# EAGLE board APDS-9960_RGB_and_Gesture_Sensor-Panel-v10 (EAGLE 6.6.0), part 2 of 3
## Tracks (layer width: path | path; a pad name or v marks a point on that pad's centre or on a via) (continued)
GND15  (via drill 0.38) (continued)
  other vias: 28.4,62.87 27.38,63.12 30.18,57.78 30.23,50.93 35.31,50.93 36.83,57.28 32.77,50.93 25.15,50.93 27.69,50.93 24.89,57.02 32.26,67.94 36.83,63.12 23.5,63.37
  pour Top (isolate 0.305): 22.61,68.83 37.85,68.83 37.85,48.51 22.61,48.51
  pour Bottom (isolate 0.305): 22.61,68.83 37.85,68.83 37.85,48.51 22.61,48.51
GND16  (via drill 0.38)
  Top 0.559: U17.6 44.76,63.27 44.76,63.25 44.42,62.92
  other vias: 44.15,62.87 43.13,63.12 45.92,57.78 45.97,50.93 51.05,50.93 52.58,57.28 48.51,50.93 40.89,50.93 43.43,50.93 40.64,57.02 48.01,67.94 52.58,63.12 39.24,63.37
  pour Top (isolate 0.305): 38.35,68.83 53.59,68.83 53.59,48.51 38.35,48.51
  pour Bottom (isolate 0.305): 38.35,68.83 53.59,68.83 53.59,48.51 38.35,48.51
GND17  (via drill 0.38)
  Top 0.559: U18.6 60.5,63.27 60.5,63.25 60.17,62.92
  other vias: 59.89,62.87 58.88,63.12 61.67,57.78 61.72,50.93 66.8,50.93 68.33,57.28 64.26,50.93 56.64,50.93 59.18,50.93 56.39,57.02 63.75,67.94 68.33,63.12 54.99,63.37
  pour Top (isolate 0.305): 54.1,68.83 69.34,68.83 69.34,48.51 54.1,48.51
  pour Bottom (isolate 0.305): 54.1,68.83 69.34,68.83 69.34,48.51 54.1,48.51
GND18  (via drill 0.38)
  Top 0.559: U19.6 76.25,63.27 76.25,63.25 75.92,62.92
  other vias: 75.64,62.87 74.63,63.12 77.42,57.78 77.47,50.93 82.55,50.93 84.07,57.28 80.01,50.93 72.39,50.93 74.93,50.93 72.14,57.02 79.5,67.94 84.07,63.12 70.74,63.37
  pour Top (isolate 0.305): 69.85,68.83 85.09,68.83 85.09,48.51 69.85,48.51
  pour Bottom (isolate 0.305): 69.85,68.83 85.09,68.83 85.09,48.51 69.85,48.51
GND19  (via drill 0.38)
  Top 0.559: 92.51,63.27 92,63.27 92,63.25 91.67,62.92
  other vias: 91.39,62.87 90.37,63.12 93.17,57.78 93.22,50.93 98.3,50.93 99.82,57.28 95.76,50.93 88.14,50.93 90.68,50.93 87.88,57.02 95.25,67.94 99.82,63.12 86.49,63.37
  pour Top (isolate 0.305): 85.6,68.83 100.84,68.83 100.84,48.51 85.6,48.51
  pour Bottom (isolate 0.305): 85.6,68.83 100.84,68.83 100.84,48.51 85.6,48.51
GND20  (via drill 0.38)
  Top 0.559: 108.25,63.27 107.75,63.27 107.75,63.25 107.42,62.92
  other vias: 107.14,62.87 106.12,63.12 108.92,57.78 108.97,50.93 114.05,50.93 115.57,57.28 111.51,50.93 103.89,50.93 106.43,50.93 103.63,57.02 111,67.94 115.57,63.12 102.23,63.37
  pour Top (isolate 0.305): 101.35,68.83 116.59,68.83 116.59,48.51 101.35,48.51
  pour Bottom (isolate 0.305): 101.35,68.83 116.59,68.83 116.59,48.51 101.35,48.51
GND21  (via drill 0.38)
  Top 0.559: 13.77,84.1 13.26,84.1 13.26,84.07 12.93,83.74
  other vias: 12.65,83.69 11.63,83.95 14.43,78.61 14.48,71.75 19.56,71.75 21.08,78.11 17.02,71.75 9.4,71.75 11.94,71.75 9.14,77.85 16.51,88.77 21.08,83.95 7.75,84.2
  pour Top (isolate 0.305): 6.86,89.66 22.1,89.66 22.1,69.34 6.86,69.34
  pour Bottom (isolate 0.305): 6.86,89.66 22.1,89.66 22.1,69.34 6.86,69.34
GND22  (via drill 0.38)
  Top 0.559: 29.52,84.1 29.01,84.1 29.01,84.07 28.68,83.74
  other vias: 28.4,83.69 27.38,83.95 30.18,78.61 30.23,71.75 35.31,71.75 36.83,78.11 32.77,71.75 25.15,71.75 27.69,71.75 24.89,77.85 32.26,88.77 36.83,83.95 23.5,84.2
  pour Top (isolate 0.305): 22.61,89.66 37.85,89.66 37.85,69.34 22.61,69.34
  pour Bottom (isolate 0.305): 22.61,89.66 37.85,89.66 37.85,69.34 22.61,69.34
GND23  (via drill 0.38)
  Top 0.559: U24.6 44.76,84.1 44.76,84.07 44.42,83.74
  other vias: 44.15,83.69 43.13,83.95 45.92,78.61 45.97,71.75 51.05,71.75 52.58,78.11 48.51,71.75 40.89,71.75 43.43,71.75 40.64,77.85 48.01,88.77 52.58,83.95 39.24,84.2
  pour Top (isolate 0.305): 38.35,89.66 53.59,89.66 53.59,69.34 38.35,69.34
  pour Bottom (isolate 0.305): 38.35,89.66 53.59,89.66 53.59,69.34 38.35,69.34
GND24  (via drill 0.38)
  Top 0.559: U25.6 60.5,84.1 60.5,84.07 60.17,83.74
  other vias: 59.89,83.69 58.88,83.95 61.67,78.61 61.72,71.75 66.8,71.75 68.33,78.11 64.26,71.75 56.64,71.75 59.18,71.75 56.39,77.85 63.75,88.77 68.33,83.95 54.99,84.2
  pour Top (isolate 0.305): 54.1,89.66 69.34,89.66 69.34,69.34 54.1,69.34
  pour Bottom (isolate 0.305): 54.1,89.66 69.34,89.66 69.34,69.34 54.1,69.34
GND25  (via drill 0.38)
  Top 0.559: U26.6 76.25,84.1 76.25,84.07 75.92,83.74
  other vias: 75.64,83.69 74.63,83.95 77.42,78.61 77.47,71.75 82.55,71.75 84.07,78.11 80.01,71.75 72.39,71.75 74.93,71.75 72.14,77.85 79.5,88.77 84.07,83.95 70.74,84.2
  pour Top (isolate 0.305): 69.85,89.66 85.09,89.66 85.09,69.34 69.85,69.34
  pour Bottom (isolate 0.305): 69.85,89.66 85.09,89.66 85.09,69.34 69.85,69.34
GND26  (via drill 0.38)
  Top 0.559: 92.51,84.1 92,84.1 92,84.07 91.67,83.74
  other vias: 91.39,83.69 90.37,83.95 93.17,78.61 93.22,71.75 98.3,71.75 99.82,78.11 95.76,71.75 88.14,71.75 90.68,71.75 87.88,77.85 95.25,88.77 99.82,83.95 86.49,84.2
  pour Top (isolate 0.305): 85.6,89.66 100.84,89.66 100.84,69.34 85.6,69.34
  pour Bottom (isolate 0.305): 85.6,89.66 100.84,89.66 100.84,69.34 85.6,69.34
GND27  (via drill 0.38)
  Top 0.559: 108.25,84.1 107.75,84.1 107.75,84.07 107.42,83.74
  other vias: 107.14,83.69 106.12,83.95 108.92,78.61 108.97,71.75 114.05,71.75 115.57,78.11 111.51,71.75 103.89,71.75 106.43,71.75 103.63,77.85 111,88.77 115.57,83.95 102.23,84.2
  pour Top (isolate 0.305): 101.35,89.66 116.59,89.66 116.59,69.34 101.35,69.34
  pour Bottom (isolate 0.305): 101.35,89.66 116.59,89.66 116.59,69.34 101.35,69.34
GND28  (via drill 0.38)
  Top 0.559: 13.77,104.93 13.26,104.93 13.26,104.9 12.93,104.57
  other vias: 12.65,104.52 11.63,104.78 14.43,99.44 14.48,92.58 19.56,92.58 21.08,98.93 17.02,92.58 9.4,92.58 11.94,92.58 9.14,98.68 16.51,109.6 21.08,104.78 7.75,105.03
  pour Top (isolate 0.305): 6.86,110.49 22.1,110.49 22.1,90.17 6.86,90.17
  pour Bottom (isolate 0.305): 6.86,110.49 22.1,110.49 22.1,90.17 6.86,90.17
GND29  (via drill 0.38)
  Top 0.559: 29.52,104.93 29.01,104.93 29.01,104.9 28.68,104.57
  other vias: 28.4,104.52 27.38,104.78 30.18,99.44 30.23,92.58 35.31,92.58 36.83,98.93 32.77,92.58 25.15,92.58 27.69,92.58 24.89,98.68 32.26,109.6 36.83,104.78 23.5,105.03
  pour Top (isolate 0.305): 22.61,110.49 37.85,110.49 37.85,90.17 22.61,90.17
  pour Bottom (isolate 0.305): 22.61,110.49 37.85,110.49 37.85,90.17 22.61,90.17
GND30  (via drill 0.38)
  Top 0.559: U31.6 44.76,104.93 44.76,104.9 44.42,104.57
  other vias: 44.15,104.52 43.13,104.78 45.92,99.44 45.97,92.58 51.05,92.58 52.58,98.93 48.51,92.58 40.89,92.58 43.43,92.58 40.64,98.68 48.01,109.6 52.58,104.78 39.24,105.03
  pour Top (isolate 0.305): 38.35,110.49 53.59,110.49 53.59,90.17 38.35,90.17
  pour Bottom (isolate 0.305): 38.35,110.49 53.59,110.49 53.59,90.17 38.35,90.17
GND31  (via drill 0.38)
  Top 0.559: U32.6 60.5,104.93 60.5,104.9 60.17,104.57
  other vias: 59.89,104.52 58.88,104.78 61.67,99.44 61.72,92.58 66.8,92.58 68.33,98.93 64.26,92.58 56.64,92.58 59.18,92.58 56.39,98.68 63.75,109.6 68.33,104.78 54.99,105.03
  pour Top (isolate 0.305): 54.1,110.49 69.34,110.49 69.34,90.17 54.1,90.17
  pour Bottom (isolate 0.305): 54.1,110.49 69.34,110.49 69.34,90.17 54.1,90.17
GND32  (via drill 0.38)
  Top 0.559: U33.6 76.25,104.93 76.25,104.9 75.92,104.57
  other vias: 75.64,104.52 74.63,104.78 77.42,99.44 77.47,92.58 82.55,92.58 84.07,98.93 80.01,92.58 72.39,92.58 74.93,92.58 72.14,98.68 79.5,109.6 84.07,104.78 70.74,105.03
  pour Top (isolate 0.305): 69.85,110.49 85.09,110.49 85.09,90.17 69.85,90.17
  pour Bottom (isolate 0.305): 69.85,110.49 85.09,110.49 85.09,90.17 69.85,90.17
GND33  (via drill 0.38)
  Top 0.559: 92.51,104.93 92,104.93 92,104.9 91.67,104.57
  other vias: 91.39,104.52 90.37,104.78 93.17,99.44 93.22,92.58 98.3,92.58 99.82,98.93 95.76,92.58 88.14,92.58 90.68,92.58 87.88,98.68 95.25,109.6 99.82,104.78 86.49,105.03
  pour Top (isolate 0.305): 85.6,110.49 100.84,110.49 100.84,90.17 85.6,90.17
  pour Bottom (isolate 0.305): 85.6,110.49 100.84,110.49 100.84,90.17 85.6,90.17
GND34  (via drill 0.38)
  Top 0.559: 108.25,104.93 107.75,104.93 107.75,104.9 107.42,104.57
  other vias: 107.14,104.52 106.12,104.78 108.92,99.44 108.97,92.58 114.05,92.58 115.57,98.93 111.51,92.58 103.89,92.58 106.43,92.58 103.63,98.68 111,109.6 115.57,104.78 102.23,105.03
  pour Top (isolate 0.305): 101.35,110.49 116.59,110.49 116.59,90.17 101.35,90.17
  pour Bottom (isolate 0.305): 101.35,110.49 116.59,110.49 116.59,90.17 101.35,90.17
INT  (via drill 0.38)
  Top 0.305: U1.2 16.28,22.58 16.51,22.35 v16.51,21.59 16.51,21.12 R1.1
  Bottom 0.305: JP1.6 20.83,14.48 18.29,17.02 18.29,19.81 v16.51,21.59
INT1  (via drill 0.38)
  Top 0.305: U2.2 32.03,22.58 32.26,22.35 v32.26,21.59 32.26,21.12 R5.1
  Bottom 0.305: JP2.6 36.58,14.48 34.04,17.02 34.04,19.81 v32.26,21.59
INT2  (via drill 0.38)
  Top 0.305: U3.2 47.77,22.58 48.01,22.35 v48.01,21.59 48.01,21.12 R9.1
  Bottom 0.305: JP3.6 52.32,14.48 49.78,17.02 49.78,19.81 v48.01,21.59
INT3  (via drill 0.38)
  Top 0.305: U4.2 63.52,22.58 63.75,22.35 v63.75,21.59 63.75,21.12 R13.1
  Bottom 0.305: JP4.6 68.07,14.48 65.53,17.02 65.53,19.81 v63.75,21.59
INT4  (via drill 0.38)
  Top 0.305: U5.2 79.27,22.58 79.5,22.35 v79.5,21.59 79.5,21.12 R17.1
  Bottom 0.305: JP5.6 83.82,14.48 81.28,17.02 81.28,19.81 v79.5,21.59
INT5  (via drill 0.38)
  Top 0.305: U6.2 95.02,22.58 95.25,22.35 v95.25,21.59 95.25,21.12 R21.1
  Bottom 0.305: JP6.6 99.57,14.48 97.03,17.02 97.03,19.81 v95.25,21.59
INT6  (via drill 0.38)
  Top 0.305: U7.2 110.77,22.58 111,22.35 v111,21.59 111,21.12 R25.1
  Bottom 0.305: JP7.6 115.32,14.48 112.78,17.02 112.78,19.81 v111,21.59
INT7  (via drill 0.38)
  Top 0.305: U8.2 16.28,43.41 16.51,43.18 v16.51,42.42 16.51,41.95 R29.1
  Bottom 0.305: JP8.6 20.83,35.31 18.29,37.85 18.29,40.64 v16.51,42.42
INT8  (via drill 0.38)
  Top 0.305: U9.2 32.03,43.41 32.26,43.18 v32.26,42.42 32.26,41.95 R33.1
  Bottom 0.305: JP9.6 36.58,35.31 34.04,37.85 34.04,40.64 v32.26,42.42
INT9  (via drill 0.38)
  Top 0.305: U10.2 47.77,43.41 48.01,43.18 v48.01,42.42 48.01,41.95 R37.1
  Bottom 0.305: JP10.6 52.32,35.31 49.78,37.85 49.78,40.64 v48.01,42.42
INT10  (via drill 0.38)
  Top 0.305: U11.2 63.52,43.41 63.75,43.18 v63.75,42.42 63.75,41.95 R41.1
  Bottom 0.305: JP11.6 68.07,35.31 65.53,37.85 65.53,40.64 v63.75,42.42
INT11  (via drill 0.38)
  Top 0.305: U12.2 79.27,43.41 79.5,43.18 v79.5,42.42 79.5,41.95 R45.1
  Bottom 0.305: JP12.6 83.82,35.31 81.28,37.85 81.28,40.64 v79.5,42.42
INT12  (via drill 0.38)
  Top 0.305: U13.2 95.02,43.41 95.25,43.18 v95.25,42.42 95.25,41.95 R49.1
  Bottom 0.305: JP13.6 99.57,35.31 97.03,37.85 97.03,40.64 v95.25,42.42
INT13  (via drill 0.38)
  Top 0.305: U14.2 110.77,43.41 111,43.18 v111,42.42 111,41.95 R53.1
  Bottom 0.305: JP14.6 115.32,35.31 112.78,37.85 112.78,40.64 v111,42.42
INT14  (via drill 0.38)
  Top 0.305: U15.2 16.28,64.24 16.51,64.01 v16.51,63.25 16.51,62.78 R57.1
  Bottom 0.305: JP15.6 20.83,56.13 18.29,58.67 18.29,61.47 v16.51,63.25
INT15  (via drill 0.38)
  Top 0.305: U16.2 32.03,64.24 32.26,64.01 v32.26,63.25 32.26,62.78 R61.1
  Bottom 0.305: JP16.6 36.58,56.13 34.04,58.67 34.04,61.47 v32.26,63.25
INT16  (via drill 0.38)
  Top 0.305: U17.2 47.77,64.24 48.01,64.01 v48.01,63.25 48.01,62.78 R65.1
  Bottom 0.305: JP17.6 52.32,56.13 49.78,58.67 49.78,61.47 v48.01,63.25
INT17  (via drill 0.38)
  Top 0.305: U18.2 63.52,64.24 63.75,64.01 v63.75,63.25 63.75,62.78 R69.1
  Bottom 0.305: JP18.6 68.07,56.13 65.53,58.67 65.53,61.47 v63.75,63.25
INT18  (via drill 0.38)
  Top 0.305: U19.2 79.27,64.24 79.5,64.01 v79.5,63.25 79.5,62.78 R73.1
  Bottom 0.305: JP19.6 83.82,56.13 81.28,58.67 81.28,61.47 v79.5,63.25
INT19  (via drill 0.38)
  Top 0.305: U20.2 95.02,64.24 95.25,64.01 v95.25,63.25 95.25,62.78 R77.1
  Bottom 0.305: JP20.6 99.57,56.13 97.03,58.67 97.03,61.47 v95.25,63.25
INT20  (via drill 0.38)
  Top 0.305: U21.2 110.77,64.24 111,64.01 v111,63.25 111,62.78 R81.1
  Bottom 0.305: JP21.6 115.32,56.13 112.78,58.67 112.78,61.47 v111,63.25
INT21  (via drill 0.38)
  Top 0.305: U22.2 16.28,85.07 16.51,84.84 v16.51,84.07 16.51,83.61 R85.1
  Bottom 0.305: JP22.6 20.83,76.96 18.29,79.5 18.29,82.3 v16.51,84.07
INT22  (via drill 0.38)
  Top 0.305: U23.2 32.03,85.07 32.26,84.84 v32.26,84.07 32.26,83.61 R89.1
  Bottom 0.305: JP23.6 36.58,76.96 34.04,79.5 34.04,82.3 v32.26,84.07
INT23  (via drill 0.38)
  Top 0.305: U24.2 47.77,85.07 48.01,84.84 v48.01,84.07 48.01,83.61 R93.1
  Bottom 0.305: JP24.6 52.32,76.96 49.78,79.5 49.78,82.3 v48.01,84.07
INT24  (via drill 0.38)
  Top 0.305: U25.2 63.52,85.07 63.75,84.84 v63.75,84.07 63.75,83.61 R97.1
  Bottom 0.305: JP25.6 68.07,76.96 65.53,79.5 65.53,82.3 v63.75,84.07
INT25  (via drill 0.38)
  Top 0.305: U26.2 79.27,85.07 79.5,84.84 v79.5,84.07 79.5,83.61 R101.1
  Bottom 0.305: JP26.6 83.82,76.96 81.28,79.5 81.28,82.3 v79.5,84.07
INT26  (via drill 0.38)
  Top 0.305: U27.2 95.02,85.07 95.25,84.84 v95.25,84.07 95.25,83.61 R105.1
  Bottom 0.305: JP27.6 99.57,76.96 97.03,79.5 97.03,82.3 v95.25,84.07
INT27  (via drill 0.38)
  Top 0.305: U28.2 110.77,85.07 111,84.84 v111,84.07 111,83.61 R109.1
  Bottom 0.305: JP28.6 115.32,76.96 112.78,79.5 112.78,82.3 v111,84.07
INT28  (via drill 0.38)
  Top 0.305: U29.2 16.28,105.89 16.51,105.66 v16.51,104.9 16.51,104.43 R113.1
  Bottom 0.305: JP29.6 20.83,97.79 18.29,100.33 18.29,103.12 v16.51,104.9
INT29  (via drill 0.38)
  Top 0.305: U30.2 32.03,105.89 32.26,105.66 v32.26,104.9 32.26,104.43 R117.1
  Bottom 0.305: JP30.6 36.58,97.79 34.04,100.33 34.04,103.12 v32.26,104.9
INT30  (via drill 0.38)
  Top 0.305: U31.2 47.77,105.89 48.01,105.66 v48.01,104.9 48.01,104.43 R121.1
  Bottom 0.305: JP31.6 52.32,97.79 49.78,100.33 49.78,103.12 v48.01,104.9
INT31  (via drill 0.38)
  Top 0.305: U32.2 63.52,105.89 63.75,105.66 v63.75,104.9 63.75,104.43 R125.1
  Bottom 0.305: JP32.6 68.07,97.79 65.53,100.33 65.53,103.12 v63.75,104.9
INT32  (via drill 0.38)
  Top 0.305: U33.2 79.27,105.89 79.5,105.66 v79.5,104.9 79.5,104.43 R129.1
  Bottom 0.305: JP33.6 83.82,97.79 81.28,100.33 81.28,103.12 v79.5,104.9
INT33  (via drill 0.38)
  Top 0.305: U34.2 95.02,105.89 95.25,105.66 v95.25,104.9 95.25,104.43 R133.1
  Bottom 0.305: JP34.6 99.57,97.79 97.03,100.33 97.03,103.12 v95.25,104.9
INT34  (via drill 0.38)
  Top 0.305: U35.2 110.77,105.89 111,105.66 v111,104.9 111,104.43 R137.1
  Bottom 0.305: JP35.6 115.32,97.79 112.78,100.33 112.78,103.12 v111,104.9
N$1
  Top 0.305: R2.2 15.75,16 16,15.75 19.3,15.75 19.56,16 19.56,16.51 19.89,16.84 SJ1.3
N$2
  Top 0.305: SJ1.1 18.32,18.47 R3.2
N$4
  Top 0.559: U1.4 U1.3
N$5
  Top 0.305: R6.2 31.5,16 31.75,15.75 35.05,15.75 35.31,16 35.31,16.51 35.64,16.84 SJ3.3
N$6
  Top 0.305: SJ3.1 34.07,18.47 R8.2
N$7
  Top 0.559: U2.4 U2.3
N$8
  Top 0.305: R10.2 47.24,16 47.5,15.75 50.8,15.75 51.05,16 51.05,16.51 51.38,16.84 SJ5.3
N$9
  Top 0.305: SJ5.1 49.82,18.47 R12.2
N$10
  Top 0.559: U3.4 U3.3
N$11
  Top 0.305: R14.2 62.99,16 63.25,15.75 66.55,15.75 66.8,16 66.8,16.51 67.13,16.84 SJ7.3
N$12
  Top 0.305: SJ7.1 65.57,18.47 R16.2
N$13
  Top 0.559: U4.4 U4.3
N$14
  Top 0.305: R18.2 78.74,16 78.99,15.75 82.3,15.75 82.55,16 82.55,16.51 82.88,16.84 SJ9.3
N$15
  Top 0.305: SJ9.1 81.32,18.47 R20.2
N$16
  Top 0.559: U5.4 U5.3
N$17
  Top 0.305: R22.2 94.49,16 94.74,15.75 98.04,15.75 98.3,16 98.3,16.51 98.63,16.84 SJ11.3
N$18
  Top 0.305: SJ11.1 97.06,18.47 R24.2
N$19
  Top 0.559: U6.4 U6.3
N$20
  Top 0.305: R26.2 110.24,16 110.49,15.75 113.79,15.75 114.05,16 114.05,16.51 114.38,16.84 SJ13.3
N$21
  Top 0.305: SJ13.1 112.81,18.47 R28.2
N$22
  Top 0.559: U7.4 U7.3
N$23
  Top 0.305: R30.2 15.75,36.83 16,36.58 19.3,36.58 19.56,36.83 19.56,37.34 19.89,37.67 SJ15.3
N$24
  Top 0.305: SJ15.1 18.32,39.29 R32.2
N$25
  Top 0.559: U8.4 U8.3
N$26
  Top 0.305: R34.2 31.5,36.83 31.75,36.58 35.05,36.58 35.31,36.83 35.31,37.34 35.64,37.67 SJ17.3
N$27
  Top 0.305: SJ17.1 34.07,39.29 R36.2
N$28
  Top 0.559: U9.4 U9.3
N$29
  Top 0.305: R38.2 47.24,36.83 47.5,36.58 50.8,36.58 51.05,36.83 51.05,37.34 51.38,37.67 SJ19.3
N$30
  Top 0.305: SJ19.1 49.82,39.29 R40.2
N$31
  Top 0.559: U10.4 U10.3
N$32
  Top 0.305: R42.2 62.99,36.83 63.25,36.58 66.55,36.58 66.8,36.83 66.8,37.34 67.13,37.67 SJ21.3
N$33
  Top 0.305: SJ21.1 65.57,39.29 R44.2
N$34
  Top 0.559: U11.4 U11.3
N$35
  Top 0.305: R46.2 78.74,36.83 78.99,36.58 82.3,36.58 82.55,36.83 82.55,37.34 82.88,37.67 SJ23.3
N$36
  Top 0.305: SJ23.1 81.32,39.29 R48.2
N$37
  Top 0.559: U12.4 U12.3
N$38
  Top 0.305: R50.2 94.49,36.83 94.74,36.58 98.04,36.58 98.3,36.83 98.3,37.34 98.63,37.67 SJ25.3
N$39
  Top 0.305: SJ25.1 97.06,39.29 R52.2
N$40
  Top 0.559: U13.4 U13.3
N$41
  Top 0.305: R54.2 110.24,36.83 110.49,36.58 113.79,36.58 114.05,36.83 114.05,37.34 114.38,37.67 SJ27.3
N$42
  Top 0.305: SJ27.1 112.81,39.29 R56.2
N$43
  Top 0.559: U14.4 U14.3
N$44
  Top 0.305: R58.2 15.75,57.66 16,57.4 19.3,57.4 19.56,57.66 19.56,58.17 19.89,58.5 SJ29.3
N$45
  Top 0.305: SJ29.1 18.32,60.12 R60.2
N$46
  Top 0.559: U15.4 U15.3
N$47
  Top 0.305: R62.2 31.5,57.66 31.75,57.4 35.05,57.4 35.31,57.66 35.31,58.17 35.64,58.5 SJ31.3
N$48
  Top 0.305: SJ31.1 34.07,60.12 R64.2
N$49
  Top 0.559: U16.4 U16.3
N$50
  Top 0.305: R66.2 47.24,57.66 47.5,57.4 50.8,57.4 51.05,57.66 51.05,58.17 51.38,58.5 SJ33.3
N$51
  Top 0.305: SJ33.1 49.82,60.12 R68.2
N$52
  Top 0.559: U17.4 U17.3
N$53
  Top 0.305: R70.2 62.99,57.66 63.25,57.4 66.55,57.4 66.8,57.66 66.8,58.17 67.13,58.5 SJ35.3
N$54
  Top 0.305: SJ35.1 65.57,60.12 R72.2
N$55
  Top 0.559: U18.4 U18.3
N$56
  Top 0.305: R74.2 78.74,57.66 78.99,57.4 82.3,57.4 82.55,57.66 82.55,58.17 82.88,58.5 SJ37.3
N$57
  Top 0.305: SJ37.1 81.32,60.12 R76.2
N$58
  Top 0.559: U19.4 U19.3
N$59
  Top 0.305: R78.2 94.49,57.66 94.74,57.4 98.04,57.4 98.3,57.66 98.3,58.17 98.63,58.5 SJ39.3
N$60
  Top 0.305: SJ39.1 97.06,60.12 R80.2
N$61
  Top 0.559: U20.4 U20.3
N$62
  Top 0.305: R82.2 110.24,57.66 110.49,57.4 113.79,57.4 114.05,57.66 114.05,58.17 114.38,58.5 SJ41.3
N$63
  Top 0.305: SJ41.1 112.81,60.12 R84.2
N$64
  Top 0.559: U21.4 U21.3
N$65
  Top 0.305: R86.2 15.75,78.49 16,78.23 19.3,78.23 19.56,78.49 19.56,78.99 19.89,79.32 SJ43.3
N$66
  Top 0.305: SJ43.1 18.32,80.95 R88.2
N$67
  Top 0.559: U22.4 U22.3
N$68
  Top 0.305: R90.2 31.5,78.49 31.75,78.23 35.05,78.23 35.31,78.49 35.31,78.99 35.64,79.32 SJ45.3
N$69
  Top 0.305: SJ45.1 34.07,80.95 R92.2
N$70
  Top 0.559: U23.4 U23.3
N$71
  Top 0.305: R94.2 47.24,78.49 47.5,78.23 50.8,78.23 51.05,78.49 51.05,78.99 51.38,79.32 SJ47.3
N$72
  Top 0.305: SJ47.1 49.82,80.95 R96.2
N$73
  Top 0.559: U24.4 U24.3
N$74
  Top 0.305: R98.2 62.99,78.49 63.25,78.23 66.55,78.23 66.8,78.49 66.8,78.99 67.13,79.32 SJ49.3
N$75
  Top 0.305: SJ49.1 65.57,80.95 R100.2
N$76
  Top 0.559: U25.4 U25.3
N$77
  Top 0.305: R102.2 78.74,78.49 78.99,78.23 82.3,78.23 82.55,78.49 82.55,78.99 82.88,79.32 SJ51.3
N$78
  Top 0.305: SJ51.1 81.32,80.95 R104.2
N$79
  Top 0.559: U26.4 U26.3
N$80
  Top 0.305: R106.2 94.49,78.49 94.74,78.23 98.04,78.23 98.3,78.49 98.3,78.99 98.63,79.32 SJ53.3
N$81
  Top 0.305: SJ53.1 97.06,80.95 R108.2
N$82
  Top 0.559: U27.4 U27.3
N$83
  Top 0.305: R110.2 110.24,78.49 110.49,78.23 113.79,78.23 114.05,78.49 114.05,78.99 114.38,79.32 SJ55.3
N$84
  Top 0.305: SJ55.1 112.81,80.95 R112.2
N$85
  Top 0.559: U28.4 U28.3
N$86
  Top 0.305: R114.2 15.75,99.31 16,99.06 19.3,99.06 19.56,99.31 19.56,99.82 19.89,100.15 SJ57.3
N$87
  Top 0.305: SJ57.1 18.32,101.78 R116.2
N$88
  Top 0.559: U29.4 U29.3
N$89
  Top 0.305: R118.2 31.5,99.31 31.75,99.06 35.05,99.06 35.31,99.31 35.31,99.82 35.64,100.15 SJ59.3
N$90
  Top 0.305: SJ59.1 34.07,101.78 R120.2
N$91
  Top 0.559: U30.4 U30.3
N$92
  Top 0.305: R122.2 47.24,99.31 47.5,99.06 50.8,99.06 51.05,99.31 51.05,99.82 51.38,100.15 SJ61.3
N$93
  Top 0.305: SJ61.1 49.82,101.78 R124.2
N$94
  Top 0.559: U31.4 U31.3
N$95
  Top 0.305: R126.2 62.99,99.31 63.25,99.06 66.55,99.06 66.8,99.31 66.8,99.82 67.13,100.15 SJ63.3
N$96
  Top 0.305: SJ63.1 65.57,101.78 R128.2
N$97
  Top 0.559: U32.4 U32.3
N$98
  Top 0.305: R130.2 78.74,99.31 78.99,99.06 82.3,99.06 82.55,99.31 82.55,99.82 82.88,100.15 SJ65.3
N$99
  Top 0.305: SJ65.1 81.32,101.78 R132.2
N$100
  Top 0.559: U33.4 U33.3
N$101
  Top 0.305: R134.2 94.49,99.31 94.74,99.06 98.04,99.06 98.3,99.31 98.3,99.82 98.63,100.15 SJ67.3
N$102
  Top 0.305: SJ67.1 97.06,101.78 R136.2
N$103
  Top 0.559: U34.4 U34.3
N$104
  Top 0.305: R138.2 110.24,99.31 110.49,99.06 113.79,99.06 114.05,99.31 114.05,99.82 114.38,100.15 SJ69.3
N$105
  Top 0.305: SJ69.1 112.81,101.78 R140.2
N$106
  Top 0.559: U35.4 U35.3
SCL  (via drill 0.38)
  Top 0.305: U1.7 12.78,22.58 v12.7,22.5 | R3.1 17.06,16.8 v17.02,16.76
  Bottom 0.305: JP1.5 18.29,15.49 v17.02,16.76 15.24,18.54 15.24,24.13 15.39,24.28 15.39,25.15 14.86,25.68 13.23,25.68 12.7,25.15 v12.7,22.5
SCL1  (via drill 0.38)
  Top 0.305: U2.7 28.53,22.58 v28.45,22.5 | R8.1 32.8,16.8 v32.77,16.76
  Bottom 0.305: JP2.5 34.04,15.49 v32.77,16.76 30.99,18.54 30.99,24.13 31.14,24.28 31.14,25.15 30.61,25.68 28.98,25.68 28.45,25.15 v28.45,22.5
SCL2  (via drill 0.38)
  Top 0.305: U3.7 44.27,22.58 v44.2,22.5 | R12.1 48.55,16.8 v48.51,16.76
  Bottom 0.305: JP3.5 49.78,15.49 v48.51,16.76 46.74,18.54 46.74,24.13 46.89,24.28 46.89,25.15 46.35,25.68 44.73,25.68 44.2,25.15 v44.2,22.5
SCL3  (via drill 0.38)
  Top 0.305: U4.7 60.02,22.58 v59.94,22.5 | R16.1 64.3,16.8 v64.26,16.76
  Bottom 0.305: JP4.5 65.53,15.49 v64.26,16.76 62.48,18.54 62.48,24.13 62.64,24.28 62.64,25.15 62.1,25.68 60.48,25.68 59.94,25.15 v59.94,22.5
SCL4  (via drill 0.38)
  Top 0.305: U5.7 75.77,22.58 v75.69,22.5 | R20.1 80.05,16.8 v80.01,16.76
  Bottom 0.305: JP5.5 81.28,15.49 v80.01,16.76 78.23,18.54 78.23,24.13 78.38,24.28 78.38,25.15 77.85,25.68 76.22,25.68 75.69,25.15 v75.69,22.5
SCL5  (via drill 0.38)
  Top 0.305: U6.7 91.52,22.58 v91.44,22.5 | R24.1 95.8,16.8 v95.76,16.76
  Bottom 0.305: JP6.5 97.03,15.49 v95.76,16.76 93.98,18.54 93.98,24.13 94.13,24.28 94.13,25.15 93.6,25.68 91.97,25.68 91.44,25.15 v91.44,22.5
SCL6  (via drill 0.38)
  Top 0.305: U7.7 107.27,22.58 v107.19,22.5 | R28.1 111.55,16.8 v111.51,16.76
  Bottom 0.305: JP7.5 112.78,15.49 v111.51,16.76 109.73,18.54 109.73,24.13 109.88,24.28 109.88,25.15 109.35,25.68 107.72,25.68 107.19,25.15 v107.19,22.5
SCL7  (via drill 0.38)
  Top 0.305: U8.7 12.78,43.41 v12.7,43.33 | R32.1 17.06,37.63 v17.02,37.59
  Bottom 0.305: JP8.5 18.29,36.32 v17.02,37.59 15.24,39.37 15.24,44.96 15.39,45.11 15.39,45.97 14.86,46.51 13.23,46.51 12.7,45.97 v12.7,43.33
SCL8  (via drill 0.38)
  Top 0.305: U9.7 28.53,43.41 v28.45,43.33 | R36.1 32.8,37.63 v32.77,37.59
  Bottom 0.305: JP9.5 34.04,36.32 v32.77,37.59 30.99,39.37 30.99,44.96 31.14,45.11 31.14,45.97 30.61,46.51 28.98,46.51 28.45,45.97 v28.45,43.33
SCL9  (via drill 0.38)
  Top 0.305: U10.7 44.27,43.41 v44.2,43.33 | R40.1 48.55,37.63 v48.51,37.59
  Bottom 0.305: JP10.5 49.78,36.32 v48.51,37.59 46.74,39.37 46.74,44.96 46.89,45.11 46.89,45.97 46.35,46.51 44.73,46.51 44.2,45.97 v44.2,43.33
SCL10  (via drill 0.38)
  Top 0.305: U11.7 60.02,43.41 v59.94,43.33 | R44.1 64.3,37.63 v64.26,37.59
  Bottom 0.305: JP11.5 65.53,36.32 v64.26,37.59 62.48,39.37 62.48,44.96 62.64,45.11 62.64,45.97 62.1,46.51 60.48,46.51 59.94,45.97 v59.94,43.33
SCL11  (via drill 0.38)
  Top 0.305: U12.7 75.77,43.41 v75.69,43.33 | R48.1 80.05,37.63 v80.01,37.59
  Bottom 0.305: JP12.5 81.28,36.32 v80.01,37.59 78.23,39.37 78.23,44.96 78.38,45.11 78.38,45.97 77.85,46.51 76.22,46.51 75.69,45.97 v75.69,43.33
SCL12  (via drill 0.38)
  Top 0.305: U13.7 91.52,43.41 v91.44,43.33 | R52.1 95.8,37.63 v95.76,37.59
  Bottom 0.305: JP13.5 97.03,36.32 v95.76,37.59 93.98,39.37 93.98,44.96 94.13,45.11 94.13,45.97 93.6,46.51 91.97,46.51 91.44,45.97 v91.44,43.33
SCL13  (via drill 0.38)
  Top 0.305: U14.7 107.27,43.41 v107.19,43.33 | R56.1 111.55,37.63 v111.51,37.59
  Bottom 0.305: JP14.5 112.78,36.32 v111.51,37.59 109.73,39.37 109.73,44.96 109.88,45.11 109.88,45.97 109.35,46.51 107.72,46.51 107.19,45.97 v107.19,43.33
SCL14  (via drill 0.38)
  Top 0.305: U15.7 12.78,64.24 v12.7,64.16 | R60.1 17.06,58.46 v17.02,58.42
  Bottom 0.305: JP15.5 18.29,57.15 v17.02,58.42 15.24,60.2 15.24,65.79 15.39,65.94 15.39,66.8 14.86,67.33 13.23,67.33 12.7,66.8 v12.7,64.16
SCL15  (via drill 0.38)
  Top 0.305: U16.7 28.53,64.24 v28.45,64.16 | R64.1 32.8,58.46 v32.77,58.42
  Bottom 0.305: JP16.5 34.04,57.15 v32.77,58.42 30.99,60.2 30.99,65.79 31.14,65.94 31.14,66.8 30.61,67.33 28.98,67.33 28.45,66.8 v28.45,64.16
SCL16  (via drill 0.38)
  Top 0.305: U17.7 44.27,64.24 v44.2,64.16 | R68.1 48.55,58.46 v48.51,58.42
  Bottom 0.305: JP17.5 49.78,57.15 v48.51,58.42 46.74,60.2 46.74,65.79 46.89,65.94 46.89,66.8 46.35,67.33 44.73,67.33 44.2,66.8 v44.2,64.16
SCL17  (via drill 0.38)
  Top 0.305: U18.7 60.02,64.24 v59.94,64.16 | R72.1 64.3,58.46 v64.26,58.42
  Bottom 0.305: JP18.5 65.53,57.15 v64.26,58.42 62.48,60.2 62.48,65.79 62.64,65.94 62.64,66.8 62.1,67.33 60.48,67.33 59.94,66.8 v59.94,64.16
SCL18  (via drill 0.38)
  Top 0.305: U19.7 75.77,64.24 v75.69,64.16 | R76.1 80.05,58.46 v80.01,58.42
  Bottom 0.305: JP19.5 81.28,57.15 v80.01,58.42 78.23,60.2 78.23,65.79 78.38,65.94 78.38,66.8 77.85,67.33 76.22,67.33 75.69,66.8 v75.69,64.16
SCL19  (via drill 0.38)
  Top 0.305: U20.7 91.52,64.24 v91.44,64.16 | R80.1 95.8,58.46 v95.76,58.42
  Bottom 0.305: JP20.5 97.03,57.15 v95.76,58.42 93.98,60.2 93.98,65.79 94.13,65.94 94.13,66.8 93.6,67.33 91.97,67.33 91.44,66.8 v91.44,64.16
SCL20  (via drill 0.38)
  Top 0.305: U21.7 107.27,64.24 v107.19,64.16 | R84.1 111.55,58.46 v111.51,58.42
  Bottom 0.305: JP21.5 112.78,57.15 v111.51,58.42 109.73,60.2 109.73,65.79 109.88,65.94 109.88,66.8 109.35,67.33 107.72,67.33 107.19,66.8 v107.19,64.16
SCL21  (via drill 0.38)
  Top 0.305: U22.7 12.78,85.07 v12.7,84.99 | R88.1 17.06,79.29 v17.02,79.25
  Bottom 0.305: JP22.5 18.29,77.98 v17.02,79.25 15.24,81.03 15.24,86.61 15.39,86.77 15.39,87.63 14.86,88.16 13.23,88.16 12.7,87.63 v12.7,84.99
SCL22  (via drill 0.38)
  Top 0.305: U23.7 28.53,85.07 v28.45,84.99 | R92.1 32.8,79.29 v32.77,79.25
  Bottom 0.305: JP23.5 34.04,77.98 v32.77,79.25 30.99,81.03 30.99,86.61 31.14,86.77 31.14,87.63 30.61,88.16 28.98,88.16 28.45,87.63 v28.45,84.99
SCL23  (via drill 0.38)
  Top 0.305: U24.7 44.27,85.07 v44.2,84.99 | R96.1 48.55,79.29 v48.51,79.25
  Bottom 0.305: JP24.5 49.78,77.98 v48.51,79.25 46.74,81.03 46.74,86.61 46.89,86.77 46.89,87.63 46.35,88.16 44.73,88.16 44.2,87.63 v44.2,84.99
SCL24  (via drill 0.38)
  Top 0.305: U25.7 60.02,85.07 v59.94,84.99 | R100.1 64.3,79.29 v64.26,79.25
  Bottom 0.305: JP25.5 65.53,77.98 v64.26,79.25 62.48,81.03 62.48,86.61 62.64,86.77 62.64,87.63 62.1,88.16 60.48,88.16 59.94,87.63 v59.94,84.99
SCL25  (via drill 0.38)
  Top 0.305: U26.7 75.77,85.07 v75.69,84.99 | R104.1 80.05,79.29 v80.01,79.25
  Bottom 0.305: JP26.5 81.28,77.98 v80.01,79.25 78.23,81.03 78.23,86.61 78.38,86.77 78.38,87.63 77.85,88.16 76.22,88.16 75.69,87.63 v75.69,84.99
SCL26  (via drill 0.38)
  Top 0.305: U27.7 91.52,85.07 v91.44,84.99 | R108.1 95.8,79.29 v95.76,79.25
  Bottom 0.305: JP27.5 97.03,77.98 v95.76,79.25 93.98,81.03 93.98,86.61 94.13,86.77 94.13,87.63 93.6,88.16 91.97,88.16 91.44,87.63 v91.44,84.99
SCL27  (via drill 0.38)
  Top 0.305: U28.7 107.27,85.07 v107.19,84.99 | R112.1 111.55,79.29 v111.51,79.25
  Bottom 0.305: JP28.5 112.78,77.98 v111.51,79.25 109.73,81.03 109.73,86.61 109.88,86.77 109.88,87.63 109.35,88.16 107.72,88.16 107.19,87.63 v107.19,84.99
SCL28  (via drill 0.38)
  Top 0.305: U29.7 12.78,105.89 v12.7,105.82 | R116.1 17.06,100.11 v17.02,100.08
  Bottom 0.305: JP29.5 18.29,98.81 v17.02,100.08 15.24,101.85 15.24,107.44 15.39,107.59 15.39,108.46 14.86,108.99 13.23,108.99 12.7,108.46 v12.7,105.82
SCL29  (via drill 0.38)
  Top 0.305: U30.7 28.53,105.89 v28.45,105.82 | R120.1 32.8,100.11 v32.77,100.08
  Bottom 0.305: JP30.5 34.04,98.81 v32.77,100.08 30.99,101.85 30.99,107.44 31.14,107.59 31.14,108.46 30.61,108.99 28.98,108.99 28.45,108.46 v28.45,105.82
SCL30  (via drill 0.38)
  Top 0.305: U31.7 44.27,105.89 v44.2,105.82 | R124.1 48.55,100.11 v48.51,100.08
  Bottom 0.305: JP31.5 49.78,98.81 v48.51,100.08 46.74,101.85 46.74,107.44 46.89,107.59 46.89,108.46 46.35,108.99 44.73,108.99 44.2,108.46 v44.2,105.82
SCL31  (via drill 0.38)
  Top 0.305: U32.7 60.02,105.89 v59.94,105.82 | R128.1 64.3,100.11 v64.26,100.08
  Bottom 0.305: JP32.5 65.53,98.81 v64.26,100.08 62.48,101.85 62.48,107.44 62.64,107.59 62.64,108.46 62.1,108.99 60.48,108.99 59.94,108.46 v59.94,105.82
SCL32  (via drill 0.38)
  Top 0.305: U33.7 75.77,105.89 v75.69,105.82 | R132.1 80.05,100.11 v80.01,100.08
  Bottom 0.305: JP33.5 81.28,98.81 v80.01,100.08 78.23,101.85 78.23,107.44 78.38,107.59 78.38,108.46 77.85,108.99 76.22,108.99 75.69,108.46 v75.69,105.82
SCL33  (via drill 0.38)
  Top 0.305: U34.7 91.52,105.89 v91.44,105.82 | R136.1 95.8,100.11 v95.76,100.08
  Bottom 0.305: JP34.5 97.03,98.81 v95.76,100.08 93.98,101.85 93.98,107.44 94.13,107.59 94.13,108.46 93.6,108.99 91.97,108.99 91.44,108.46 v91.44,105.82
SCL34  (via drill 0.38)
  Top 0.305: U35.7 107.27,105.89 v107.19,105.82 | R140.1 111.55,100.11 v111.51,100.08
  Bottom 0.305: JP35.5 112.78,98.81 v111.51,100.08 109.73,101.85 109.73,107.44 109.88,107.59 109.88,108.46 109.35,108.99 107.72,108.99 107.19,108.46 v107.19,105.82
SDA  (via drill 0.38)
  Top 0.305: v14.48,17.65 14.48,18.29 14.69,18.5 R2.1 | U1.1 15.18,24.19 14.61,24.77 v14.48,24.77
  Bottom 0.305: v14.48,24.77 v14.48,17.65 15.75,16.38 JP1.4
SDA1  (via drill 0.38)
  Top 0.305: v30.23,17.65 30.23,18.29 30.44,18.5 R6.1 | U2.1 30.93,24.19 30.35,24.77 v30.23,24.77
  Bottom 0.305: v30.23,24.77 v30.23,17.65 31.5,16.38 JP2.4
SDA2  (via drill 0.38)
  Top 0.305: v45.97,17.65 45.97,18.29 46.19,18.5 R10.1 | U3.1 46.67,24.19 46.1,24.77 v45.97,24.77
  Bottom 0.305: v45.97,24.77 v45.97,17.65 47.24,16.38 JP3.4
SDA3  (via drill 0.38)
  Top 0.305: v61.72,17.65 61.72,18.29 61.94,18.5 R14.1 | U4.1 62.42,24.19 61.85,24.77 v61.72,24.77
  Bottom 0.305: v61.72,24.77 v61.72,17.65 62.99,16.38 JP4.4
SDA4  (via drill 0.38)
  Top 0.305: v77.47,17.65 77.47,18.29 77.69,18.5 R18.1 | U5.1 78.17,24.19 77.6,24.77 v77.47,24.77
  Bottom 0.305: v77.47,24.77 v77.47,17.65 78.74,16.38 JP5.4
SDA5  (via drill 0.38)
  Top 0.305: v93.22,17.65 93.22,18.29 93.43,18.5 R22.1 | U6.1 93.92,24.19 93.34,24.77 v93.22,24.77
  Bottom 0.305: v93.22,24.77 v93.22,17.65 94.49,16.38 JP6.4
SDA6  (via drill 0.38)
  Top 0.305: v108.97,17.65 108.97,18.29 109.18,18.5 R26.1 | U7.1 109.67,24.19 109.09,24.77 v108.97,24.77
  Bottom 0.305: v108.97,24.77 v108.97,17.65 110.24,16.38 JP7.4
SDA7  (via drill 0.38)
  Top 0.305: v14.48,38.48 14.48,39.12 14.69,39.33 R30.1 | U8.1 15.18,45.02 14.61,45.59 v14.48,45.59
  Bottom 0.305: v14.48,45.59 v14.48,38.48 15.75,37.21 JP8.4
SDA8  (via drill 0.38)
  Top 0.305: v30.23,38.48 30.23,39.12 30.44,39.33 R34.1 | U9.1 30.93,45.02 30.35,45.59 v30.23,45.59
  Bottom 0.305: v30.23,45.59 v30.23,38.48 31.5,37.21 JP9.4
SDA9  (via drill 0.38)
  Top 0.305: v45.97,38.48 45.97,39.12 46.19,39.33 R38.1 | U10.1 46.67,45.02 46.1,45.59 v45.97,45.59
  Bottom 0.305: v45.97,45.59 v45.97,38.48 47.24,37.21 JP10.4
SDA10  (via drill 0.38)
  Top 0.305: v61.72,38.48 61.72,39.12 61.94,39.33 R42.1 | U11.1 62.42,45.02 61.85,45.59 v61.72,45.59
  Bottom 0.305: v61.72,45.59 v61.72,38.48 62.99,37.21 JP11.4
SDA11  (via drill 0.38)
  Top 0.305: v77.47,38.48 77.47,39.12 77.69,39.33 R46.1 | U12.1 78.17,45.02 77.6,45.59 v77.47,45.59
  Bottom 0.305: v77.47,45.59 v77.47,38.48 78.74,37.21 JP12.4
SDA12  (via drill 0.38)
  Top 0.305: v93.22,38.48 93.22,39.12 93.43,39.33 R50.1 | U13.1 93.92,45.02 93.34,45.59 v93.22,45.59
  Bottom 0.305: v93.22,45.59 v93.22,38.48 94.49,37.21 JP13.4
SDA13  (via drill 0.38)
  Top 0.305: v108.97,38.48 108.97,39.12 109.18,39.33 R54.1 | U14.1 109.67,45.02 109.09,45.59 v108.97,45.59
  Bottom 0.305: v108.97,45.59 v108.97,38.48 110.24,37.21 JP14.4
SDA14  (via drill 0.38)
  Top 0.305: v14.48,59.31 14.48,59.94 14.69,60.16 R58.1 | U15.1 15.18,65.85 14.61,66.42 v14.48,66.42
  Bottom 0.305: v14.48,66.42 v14.48,59.31 15.75,58.04 JP15.4
SDA15  (via drill 0.38)
  Top 0.305: v30.23,59.31 30.23,59.94 30.44,60.16 R62.1 | U16.1 30.93,65.85 30.35,66.42 v30.23,66.42
  Bottom 0.305: v30.23,66.42 v30.23,59.31 31.5,58.04 JP16.4
SDA16  (via drill 0.38)
  Top 0.305: v45.97,59.31 45.97,59.94 46.19,60.16 R66.1 | U17.1 46.67,65.85 46.1,66.42 v45.97,66.42
  Bottom 0.305: v45.97,66.42 v45.97,59.31 47.24,58.04 JP17.4
SDA17  (via drill 0.38)
  Top 0.305: v61.72,59.31 61.72,59.94 61.94,60.16 R70.1 | U18.1 62.42,65.85 61.85,66.42 v61.72,66.42
  Bottom 0.305: v61.72,66.42 v61.72,59.31 62.99,58.04 JP18.4
SDA18  (via drill 0.38)
  Top 0.305: v77.47,59.31 77.47,59.94 77.69,60.16 R74.1 | U19.1 78.17,65.85 77.6,66.42 v77.47,66.42
  Bottom 0.305: v77.47,66.42 v77.47,59.31 78.74,58.04 JP19.4
SDA19  (via drill 0.38)
  Top 0.305: v93.22,59.31 93.22,59.94 93.43,60.16 R78.1 | U20.1 93.92,65.85 93.34,66.42 v93.22,66.42
  Bottom 0.305: v93.22,66.42 v93.22,59.31 94.49,58.04 JP20.4
SDA20  (via drill 0.38)
  Top 0.305: v108.97,59.31 108.97,59.94 109.18,60.16 R82.1 | U21.1 109.67,65.85 109.09,66.42 v108.97,66.42
  Bottom 0.305: v108.97,66.42 v108.97,59.31 110.24,58.04 JP21.4
SDA21  (via drill 0.38)
  Top 0.305: v14.48,80.14 14.48,80.77 14.69,80.99 R86.1 | U22.1 15.18,86.68 14.61,87.25 v14.48,87.25
  Bottom 0.305: v14.48,87.25 v14.48,80.14 15.75,78.87 JP22.4
SDA22  (via drill 0.38)
  Top 0.305: v30.23,80.14 30.23,80.77 30.44,80.99 R90.1 | U23.1 30.93,86.68 30.35,87.25 v30.23,87.25
  Bottom 0.305: v30.23,87.25 v30.23,80.14 31.5,78.87 JP23.4
SDA23  (via drill 0.38)
  Top 0.305: v45.97,80.14 45.97,80.77 46.19,80.99 R94.1 | U24.1 46.67,86.68 46.1,87.25 v45.97,87.25
  Bottom 0.305: v45.97,87.25 v45.97,80.14 47.24,78.87 JP24.4
SDA24  (via drill 0.38)
  Top 0.305: v61.72,80.14 61.72,80.77 61.94,80.99 R98.1 | U25.1 62.42,86.68 61.85,87.25 v61.72,87.25
  Bottom 0.305: v61.72,87.25 v61.72,80.14 62.99,78.87 JP25.4
SDA25  (via drill 0.38)
  Top 0.305: v77.47,80.14 77.47,80.77 77.69,80.99 R102.1 | U26.1 78.17,86.68 77.6,87.25 v77.47,87.25
  Bottom 0.305: v77.47,87.25 v77.47,80.14 78.74,78.87 JP26.4
SDA26  (via drill 0.38)
  Top 0.305: v93.22,80.14 93.22,80.77 93.43,80.99 R106.1 | U27.1 93.92,86.68 93.34,87.25 v93.22,87.25
  Bottom 0.305: v93.22,87.25 v93.22,80.14 94.49,78.87 JP27.4
SDA27  (via drill 0.38)
  Top 0.305: v108.97,80.14 108.97,80.77 109.18,80.99 R110.1 | U28.1 109.67,86.68 109.09,87.25 v108.97,87.25
  Bottom 0.305: v108.97,87.25 v108.97,80.14 110.24,78.87 JP28.4
SDA28  (via drill 0.38)
  Top 0.305: v14.48,100.97 14.48,101.6 14.69,101.81 R114.1 | U29.1 15.18,107.5 14.61,108.08 v14.48,108.08
  Bottom 0.305: v14.48,108.08 v14.48,100.97 15.75,99.69 JP29.4
SDA29  (via drill 0.38)
  Top 0.305: v30.23,100.97 30.23,101.6 30.44,101.81 R118.1 | U30.1 30.93,107.5 30.35,108.08 v30.23,108.08
  Bottom 0.305: v30.23,108.08 v30.23,100.97 31.5,99.69 JP30.4
SDA30  (via drill 0.38)
  Top 0.305: v45.97,100.97 45.97,101.6 46.19,101.81 R122.1 | U31.1 46.67,107.5 46.1,108.08 v45.97,108.08
  Bottom 0.305: v45.97,108.08 v45.97,100.97 47.24,99.69 JP31.4
SDA31  (via drill 0.38)
  Top 0.305: v61.72,100.97 61.72,101.6 61.94,101.81 R126.1 | U32.1 62.42,107.5 61.85,108.08 v61.72,108.08
  Bottom 0.305: v61.72,108.08 v61.72,100.97 62.99,99.69 JP32.4
SDA32  (via drill 0.38)
  Top 0.305: v77.47,100.97 77.47,101.6 77.69,101.81 R130.1 | U33.1 78.17,107.5 77.6,108.08 v77.47,108.08
  Bottom 0.305: v77.47,108.08 v77.47,100.97 78.74,99.69 JP33.4
SDA33  (via drill 0.38)
  Top 0.305: v93.22,100.97 93.22,101.6 93.43,101.81 R134.1 | U34.1 93.92,107.5 93.34,108.08 v93.22,108.08
  Bottom 0.305: v93.22,108.08 v93.22,100.97 94.49,99.69 JP34.4
SDA34  (via drill 0.38)
  Top 0.305: v108.97,100.97 108.97,101.6 109.18,101.81 R138.1 | U35.1 109.67,107.5 109.09,108.08 v108.97,108.08
  Bottom 0.305: v108.97,108.08 v108.97,100.97 110.24,99.69 JP35.4
VCC  (via drill 0.38)
  Top 0.305: SJ1.2 v19.56,17.65 | v20.57,20.19 R1.2 19.14,20.99 18.8,21.34 18.29,21.34 16,23.62 16,24.64 14.99,25.65 13.97,25.65 12.7,24.38 12.7,23.55
  Top 0.559: 9.61,18.5 9.18,18.07 SJ2.2 8.13,18.26 | R4.2 9.61,18.5 | 9.61,18.5 9.61,19.27 9.82,19.47 C3.1 9.82,21.25 12.12,23.55 12.7,23.55 U1.8
  Top 0.762: 8.13,18.26 v8.13,19.56 v8.13,20.57
  Bottom 0.305: v20.57,20.19 20.57,18.67 v19.56,17.65
  Bottom 0.762: v8.13,20.57 v8.13,19.56 8.13,18.8 13.21,13.72 JP1.3
VCC1  (via drill 0.38)
  Top 0.305: SJ3.2 v35.31,17.65 | v36.32,20.19 R5.2 34.89,20.99 34.54,21.34 34.04,21.34 31.75,23.62 31.75,24.64 30.73,25.65 29.72,25.65 28.45,24.38 28.45,23.55
  Top 0.559: 25.36,18.5 24.92,18.07 SJ4.2 23.88,18.26 | R7.2 25.36,18.5 | 25.36,18.5 25.36,19.27 25.57,19.47 C5.1 25.57,21.25 27.87,23.55 28.45,23.55 U2.8
  Top 0.762: 23.88,18.26 v23.88,19.56 v23.88,20.57
  Bottom 0.305: v36.32,20.19 36.32,18.67 v35.31,17.65
  Bottom 0.762: v23.88,20.57 v23.88,19.56 23.88,18.8 28.96,13.72 JP2.3
VCC2  (via drill 0.38)
  Top 0.305: SJ5.2 v51.05,17.65 | v52.07,20.19 R9.2 50.63,20.99 50.29,21.34 49.78,21.34 47.5,23.62 47.5,24.64 46.48,25.65 45.47,25.65 44.2,24.38 44.2,23.55
  Top 0.559: 41.11,18.5 40.67,18.07 SJ6.2 39.62,18.26 | R11.2 41.11,18.5 | 41.11,18.5 41.11,19.27 41.31,19.47 C8.1 41.31,21.25 43.62,23.55 44.2,23.55 U3.8
  Top 0.762: 39.62,18.26 v39.62,19.56 v39.62,20.57
  Bottom 0.305: v52.07,20.19 52.07,18.67 v51.05,17.65
  Bottom 0.762: v39.62,20.57 v39.62,19.56 39.62,18.8 44.7,13.72 JP3.3
VCC3  (via drill 0.38)
  Top 0.305: SJ7.2 v66.8,17.65 | v67.82,20.19 R13.2 66.38,20.99 66.04,21.34 65.53,21.34 63.25,23.62 63.25,24.64 62.23,25.65 61.21,25.65 59.94,24.38 59.94,23.55
  Top 0.559: 56.86,18.5 56.42,18.07 SJ8.2 55.37,18.26 | R15.2 56.86,18.5 | 56.86,18.5 56.86,19.27 57.06,19.47 C11.1 57.06,21.25 59.37,23.55 59.94,23.55 U4.8
  Top 0.762: 55.37,18.26 v55.37,19.56 v55.37,20.57
  Bottom 0.305: v67.82,20.19 67.82,18.67 v66.8,17.65
  Bottom 0.762: v55.37,20.57 v55.37,19.56 55.37,18.8 60.45,13.72 JP4.3
VCC4  (via drill 0.38)
  Top 0.305: SJ9.2 v82.55,17.65 | v83.57,20.19 R17.2 82.13,20.99 81.79,21.34 81.28,21.34 78.99,23.62 78.99,24.64 77.98,25.65 76.96,25.65 75.69,24.38 75.69,23.55
  Top 0.559: 72.61,18.5 72.17,18.07 SJ10.2 71.12,18.26 | R19.2 72.61,18.5 | 72.61,18.5 72.61,19.27 72.81,19.47 C14.1 72.81,21.25 75.11,23.55 75.69,23.55 U5.8
  Top 0.762: 71.12,18.26 v71.12,19.56 v71.12,20.57
  Bottom 0.305: v83.57,20.19 83.57,18.67 v82.55,17.65
  Bottom 0.762: v71.12,20.57 v71.12,19.56 71.12,18.8 76.2,13.72 JP5.3
VCC5  (via drill 0.38)
  Top 0.305: SJ11.2 v98.3,17.65 | v99.31,20.19 R21.2 97.88,20.99 97.54,21.34 97.03,21.34 94.74,23.62 94.74,24.64 93.73,25.65 92.71,25.65 91.44,24.38 91.44,23.55
  Top 0.559: 88.35,18.5 87.92,18.07 SJ12.2 86.87,18.26 | R23.2 88.35,18.5 | 88.35,18.5 88.35,19.27 88.56,19.47 C17.1 88.56,21.25 90.86,23.55 91.44,23.55 U6.8
  Top 0.762: 86.87,18.26 v86.87,19.56 v86.87,20.57
  Bottom 0.305: v99.31,20.19 99.31,18.67 v98.3,17.65
  Bottom 0.762: v86.87,20.57 v86.87,19.56 86.87,18.8 91.95,13.72 JP6.3
VCC6  (via drill 0.38)
  Top 0.305: SJ13.2 v114.05,17.65 | v115.06,20.19 R25.2 113.63,20.99 113.28,21.34 112.78,21.34 110.49,23.62 110.49,24.64 109.47,25.65 108.46,25.65 107.19,24.38 107.19,23.55
  Top 0.559: 104.1,18.5 103.66,18.07 SJ14.2 102.62,18.26 | R27.2 104.1,18.5 | 104.1,18.5 104.1,19.27 104.31,19.47 C20.1 104.31,21.25 106.61,23.55 107.19,23.55 U7.8
  Top 0.762: 102.62,18.26 v102.62,19.56 v102.62,20.57
  Bottom 0.305: v115.06,20.19 115.06,18.67 v114.05,17.65
  Bottom 0.762: v102.62,20.57 v102.62,19.56 102.62,18.8 107.7,13.72 JP7.3
VCC7  (via drill 0.38)
  Top 0.305: SJ15.2 v19.56,38.48 | v20.57,41.02 R29.2 19.14,41.82 18.8,42.16 18.29,42.16 16,44.45 16,45.47 14.99,46.48 13.97,46.48 12.7,45.21 12.7,44.38
  Top 0.559: 9.61,39.33 9.18,38.89 SJ16.2 8.13,39.09 | R31.2 9.61,39.33 | 9.61,39.33 9.61,40.09 9.82,40.3 C23.1 9.82,42.08 12.12,44.38 12.7,44.38 U8.8
  Top 0.762: 8.13,39.09 v8.13,40.39 v8.13,41.4
  Bottom 0.305: v20.57,41.02 20.57,39.5 v19.56,38.48
  Bottom 0.762: v8.13,41.4 v8.13,40.39 8.13,39.62 13.21,34.54 JP8.3
VCC8  (via drill 0.38)
  Top 0.305: SJ17.2 v35.31,38.48 | v36.32,41.02 R33.2 34.89,41.82 34.54,42.16 34.04,42.16 31.75,44.45 31.75,45.47 30.73,46.48 29.72,46.48 28.45,45.21 28.45,44.38
  Top 0.559: 25.36,39.33 24.92,38.89 SJ18.2 23.88,39.09 | R35.2 25.36,39.33 | 25.36,39.33 25.36,40.09 25.57,40.3 C26.1 25.57,42.08 27.87,44.38 28.45,44.38 U9.8
  Top 0.762: 23.88,39.09 v23.88,40.39 v23.88,41.4
  Bottom 0.305: v36.32,41.02 36.32,39.5 v35.31,38.48
  Bottom 0.762: v23.88,41.4 v23.88,40.39 23.88,39.62 28.96,34.54 JP9.3
VCC9  (via drill 0.38)
  Top 0.305: SJ19.2 v51.05,38.48 | v52.07,41.02 R37.2 50.63,41.82 50.29,42.16 49.78,42.16 47.5,44.45 47.5,45.47 46.48,46.48 45.47,46.48 44.2,45.21 44.2,44.38
  Top 0.559: 41.11,39.33 40.67,38.89 SJ20.2 39.62,39.09 | R39.2 41.11,39.33 | 41.11,39.33 41.11,40.09 41.31,40.3 C29.1 41.31,42.08 43.62,44.38 44.2,44.38 U10.8
  Top 0.762: 39.62,39.09 v39.62,40.39 v39.62,41.4
  Bottom 0.305: v52.07,41.02 52.07,39.5 v51.05,38.48
  Bottom 0.762: v39.62,41.4 v39.62,40.39 39.62,39.62 44.7,34.54 JP10.3
VCC10  (via drill 0.38)
  Top 0.305: SJ21.2 v66.8,38.48 | v67.82,41.02 R41.2 66.38,41.82 66.04,42.16 65.53,42.16 63.25,44.45 63.25,45.47 62.23,46.48 61.21,46.48 59.94,45.21 59.94,44.38
  Top 0.559: 56.86,39.33 56.42,38.89 SJ22.2 55.37,39.09 | R43.2 56.86,39.33 | 56.86,39.33 56.86,40.09 57.06,40.3 C32.1 57.06,42.08 59.37,44.38 59.94,44.38 U11.8
  Top 0.762: 55.37,39.09 v55.37,40.39 v55.37,41.4
  Bottom 0.305: v67.82,41.02 67.82,39.5 v66.8,38.48
  Bottom 0.762: v55.37,41.4 v55.37,40.39 55.37,39.62 60.45,34.54 JP11.3
VCC11  (via drill 0.38)
  Top 0.305: SJ23.2 v82.55,38.48 | v83.57,41.02 R45.2 82.13,41.82 81.79,42.16 81.28,42.16 78.99,44.45 78.99,45.47 77.98,46.48 76.96,46.48 75.69,45.21 75.69,44.38
  Top 0.559: 72.61,39.33 72.17,38.89 SJ24.2 71.12,39.09 | R47.2 72.61,39.33 | 72.61,39.33 72.61,40.09 72.81,40.3 C35.1 72.81,42.08 75.11,44.38 75.69,44.38 U12.8
  Top 0.762: 71.12,39.09 v71.12,40.39 v71.12,41.4
  Bottom 0.305: v83.57,41.02 83.57,39.5 v82.55,38.48
  Bottom 0.762: v71.12,41.4 v71.12,40.39 71.12,39.62 76.2,34.54 JP12.3
VCC12  (via drill 0.38)
  Top 0.305: SJ25.2 v98.3,38.48 | v99.31,41.02 R49.2 97.88,41.82 97.54,42.16 97.03,42.16 94.74,44.45 94.74,45.47 93.73,46.48 92.71,46.48 91.44,45.21 91.44,44.38
  Top 0.559: 88.35,39.33 87.92,38.89 SJ26.2 86.87,39.09 | R51.2 88.35,39.33 | 88.35,39.33 88.35,40.09 88.56,40.3 C38.1 88.56,42.08 90.86,44.38 91.44,44.38 U13.8
  Top 0.762: 86.87,39.09 v86.87,40.39 v86.87,41.4
  Bottom 0.305: v99.31,41.02 99.31,39.5 v98.3,38.48
  Bottom 0.762: v86.87,41.4 v86.87,40.39 86.87,39.62 91.95,34.54 JP13.3
VCC13  (via drill 0.38)
  Top 0.305: SJ27.2 v114.05,38.48 | v115.06,41.02 R53.2 113.63,41.82 113.28,42.16 112.78,42.16 110.49,44.45 110.49,45.47 109.47,46.48 108.46,46.48 107.19,45.21 107.19,44.38
  Top 0.559: 104.1,39.33 103.66,38.89 SJ28.2 102.62,39.09 | R55.2 104.1,39.33 | 104.1,39.33 104.1,40.09 104.31,40.3 C41.1 104.31,42.08 106.61,44.38 107.19,44.38 U14.8
  Top 0.762: 102.62,39.09 v102.62,40.39 v102.62,41.4
  Bottom 0.305: v115.06,41.02 115.06,39.5 v114.05,38.48
  Bottom 0.762: v102.62,41.4 v102.62,40.39 102.62,39.62 107.7,34.54 JP14.3
VCC14  (via drill 0.38)
  Top 0.305: SJ29.2 v19.56,59.31 | v20.57,61.85 R57.2 19.14,62.65 18.8,62.99 18.29,62.99 16,65.28 16,66.29 14.99,67.31 13.97,67.31 12.7,66.04 12.7,65.21
  Top 0.559: 9.61,60.16 9.18,59.72 SJ30.2 8.13,59.92 | R59.2 9.61,60.16 | 9.61,60.16 9.61,60.92 9.82,61.13 C44.1 9.82,62.9 12.12,65.21 12.7,65.21 U15.8
  Top 0.762: 8.13,59.92 v8.13,61.21 v8.13,62.23
  Bottom 0.305: v20.57,61.85 20.57,60.33 v19.56,59.31
  Bottom 0.762: v8.13,62.23 v8.13,61.21 8.13,60.45 13.21,55.37 JP15.3
VCC15  (via drill 0.38)
  Top 0.305: SJ31.2 v35.31,59.31 | v36.32,61.85 R61.2 34.89,62.65 34.54,62.99 34.04,62.99 31.75,65.28 31.75,66.29 30.73,67.31 29.72,67.31 28.45,66.04 28.45,65.21
  Top 0.559: 25.36,60.16 24.92,59.72 SJ32.2 23.88,59.92 | R63.2 25.36,60.16 | 25.36,60.16 25.36,60.92 25.57,61.13 C47.1 25.57,62.9 27.87,65.21 28.45,65.21 U16.8
  Top 0.762: 23.88,59.92 v23.88,61.21 v23.88,62.23
  Bottom 0.305: v36.32,61.85 36.32,60.33 v35.31,59.31
  Bottom 0.762: v23.88,62.23 v23.88,61.21 23.88,60.45 28.96,55.37 JP16.3
VCC16  (via drill 0.38)
  Top 0.305: SJ33.2 v51.05,59.31 | v52.07,61.85 R65.2 50.63,62.65 50.29,62.99 49.78,62.99 47.5,65.28 47.5,66.29 46.48,67.31 45.47,67.31 44.2,66.04 44.2,65.21
  Top 0.559: 41.11,60.16 40.67,59.72 SJ34.2 39.62,59.92 | R67.2 41.11,60.16 | 41.11,60.16 41.11,60.92 41.31,61.13 C50.1 41.31,62.9 43.62,65.21 44.2,65.21 U17.8
  Top 0.762: 39.62,59.92 v39.62,61.21 v39.62,62.23
  Bottom 0.305: v52.07,61.85 52.07,60.33 v51.05,59.31
  Bottom 0.762: v39.62,62.23 v39.62,61.21 39.62,60.45 44.7,55.37 JP17.3
VCC17  (via drill 0.38)
  Top 0.305: SJ35.2 v66.8,59.31 | v67.82,61.85 R69.2 66.38,62.65 66.04,62.99 65.53,62.99 63.25,65.28 63.25,66.29 62.23,67.31 61.21,67.31 59.94,66.04 59.94,65.21
  Top 0.559: 56.86,60.16 56.42,59.72 SJ36.2 55.37,59.92 | R71.2 56.86,60.16 | 56.86,60.16 56.86,60.92 57.06,61.13 C53.1 57.06,62.9 59.37,65.21 59.94,65.21 U18.8
  Top 0.762: 55.37,59.92 v55.37,61.21 v55.37,62.23
  Bottom 0.305: v67.82,61.85 67.82,60.33 v66.8,59.31
  Bottom 0.762: v55.37,62.23 v55.37,61.21 55.37,60.45 60.45,55.37 JP18.3
VCC18  (via drill 0.38)
  Top 0.305: SJ37.2 v82.55,59.31 | v83.57,61.85 R73.2 82.13,62.65 81.79,62.99 81.28,62.99 78.99,65.28 78.99,66.29 77.98,67.31 76.96,67.31 75.69,66.04 75.69,65.21
  Top 0.559: 72.61,60.16 72.17,59.72 SJ38.2 71.12,59.92 | R75.2 72.61,60.16 | 72.61,60.16 72.61,60.92 72.81,61.13 C56.1 72.81,62.9 75.11,65.21 75.69,65.21 U19.8
  Top 0.762: 71.12,59.92 v71.12,61.21 v71.12,62.23
  Bottom 0.305: v83.57,61.85 83.57,60.33 v82.55,59.31
  Bottom 0.762: v71.12,62.23 v71.12,61.21 71.12,60.45 76.2,55.37 JP19.3
VCC19  (via drill 0.38)
  Top 0.305: SJ39.2 v98.3,59.31 | v99.31,61.85 R77.2 97.88,62.65 97.54,62.99 97.03,62.99 94.74,65.28 94.74,66.29 93.73,67.31 92.71,67.31 91.44,66.04 91.44,65.21
  Top 0.559: 88.35,60.16 87.92,59.72 SJ40.2 86.87,59.92 | R79.2 88.35,60.16 | 88.35,60.16 88.35,60.92 88.56,61.13 C59.1 88.56,62.9 90.86,65.21 91.44,65.21 U20.8
  Top 0.762: 86.87,59.92 v86.87,61.21 v86.87,62.23
  Bottom 0.305: v99.31,61.85 99.31,60.33 v98.3,59.31
  Bottom 0.762: v86.87,62.23 v86.87,61.21 86.87,60.45 91.95,55.37 JP20.3
VCC20  (via drill 0.38)
  Top 0.305: SJ41.2 v114.05,59.31 | v115.06,61.85 R81.2 113.63,62.65 113.28,62.99 112.78,62.99 110.49,65.28 110.49,66.29 109.47,67.31 108.46,67.31 107.19,66.04 107.19,65.21
  Top 0.559: 104.1,60.16 103.66,59.72 SJ42.2 102.62,59.92 | R83.2 104.1,60.16 | 104.1,60.16 104.1,60.92 104.31,61.13 C62.1 104.31,62.9 106.61,65.21 107.19,65.21 U21.8
  Top 0.762: 102.62,59.92 v102.62,61.21 v102.62,62.23
  Bottom 0.305: v115.06,61.85 115.06,60.33 v114.05,59.31
  Bottom 0.762: v102.62,62.23 v102.62,61.21 102.62,60.45 107.7,55.37 JP21.3
VCC21  (via drill 0.38)
  Top 0.305: SJ43.2 v19.56,80.14 | v20.57,82.68 R85.2 19.14,83.48 18.8,83.82 18.29,83.82 16,86.11 16,87.12 14.99,88.14 13.97,88.14 12.7,86.87 12.7,86.04
  Top 0.559: 9.61,80.99 9.18,80.55 SJ44.2 8.13,80.75 | R87.2 9.61,80.99 | 9.61,80.99 9.61,81.75 9.82,81.95 C65.1 9.82,83.73 12.12,86.04 12.7,86.04 U22.8
  Top 0.762: 8.13,80.75 v8.13,82.04 v8.13,83.06
  Bottom 0.305: v20.57,82.68 20.57,81.15 v19.56,80.14
  Bottom 0.762: v8.13,83.06 v8.13,82.04 8.13,81.28 13.21,76.2 JP22.3
VCC22  (via drill 0.38)
  Top 0.305: SJ45.2 v35.31,80.14 | v36.32,82.68 R89.2 34.89,83.48 34.54,83.82 34.04,83.82 31.75,86.11 31.75,87.12 30.73,88.14 29.72,88.14 28.45,86.87 28.45,86.04
  Top 0.559: 25.36,80.99 24.92,80.55 SJ46.2 23.88,80.75 | R91.2 25.36,80.99 | 25.36,80.99 25.36,81.75 25.57,81.95 C68.1 25.57,83.73 27.87,86.04 28.45,86.04 U23.8
  Top 0.762: 23.88,80.75 v23.88,82.04 v23.88,83.06
  Bottom 0.305: v36.32,82.68 36.32,81.15 v35.31,80.14
  Bottom 0.762: v23.88,83.06 v23.88,82.04 23.88,81.28 28.96,76.2 JP23.3
VCC23  (via drill 0.38)
  Top 0.305: SJ47.2 v51.05,80.14 | v52.07,82.68 R93.2 50.63,83.48 50.29,83.82 49.78,83.82 47.5,86.11 47.5,87.12 46.48,88.14 45.47,88.14 44.2,86.87 44.2,86.04
  Top 0.559: 41.11,80.99 40.67,80.55 SJ48.2 39.62,80.75 | R95.2 41.11,80.99 | 41.11,80.99 41.11,81.75 41.31,81.95 C71.1 41.31,83.73 43.62,86.04 44.2,86.04 U24.8
  Top 0.762: 39.62,80.75 v39.62,82.04 v39.62,83.06
  Bottom 0.305: v52.07,82.68 52.07,81.15 v51.05,80.14
  Bottom 0.762: v39.62,83.06 v39.62,82.04 39.62,81.28 44.7,76.2 JP24.3
VCC24  (via drill 0.38)
  Top 0.305: SJ49.2 v66.8,80.14 | v67.82,82.68 R97.2 66.38,83.48 66.04,83.82 65.53,83.82 63.25,86.11 63.25,87.12 62.23,88.14 61.21,88.14 59.94,86.87 59.94,86.04
  Top 0.559: 56.86,80.99 56.42,80.55 SJ50.2 55.37,80.75 | R99.2 56.86,80.99 | 56.86,80.99 56.86,81.75 57.06,81.95 C74.1 57.06,83.73 59.37,86.04 59.94,86.04 U25.8
  Top 0.762: 55.37,80.75 v55.37,82.04 v55.37,83.06
  Bottom 0.305: v67.82,82.68 67.82,81.15 v66.8,80.14
  Bottom 0.762: v55.37,83.06 v55.37,82.04 55.37,81.28 60.45,76.2 JP25.3
VCC25  (via drill 0.38)
  Top 0.305: SJ51.2 v82.55,80.14 | v83.57,82.68 R101.2 82.13,83.48 81.79,83.82 81.28,83.82 78.99,86.11 78.99,87.12 77.98,88.14 76.96,88.14 75.69,86.87 75.69,86.04
  Top 0.559: 72.61,80.99 72.17,80.55 SJ52.2 71.12,80.75 | R103.2 72.61,80.99 | 72.61,80.99 72.61,81.75 72.81,81.95 C77.1 72.81,83.73 75.11,86.04 75.69,86.04 U26.8
  Top 0.762: 71.12,80.75 v71.12,82.04 v71.12,83.06
  Bottom 0.305: v83.57,82.68 83.57,81.15 v82.55,80.14
  Bottom 0.762: v71.12,83.06 v71.12,82.04 71.12,81.28 76.2,76.2 JP26.3
VCC26  (via drill 0.38)
  Top 0.305: SJ53.2 v98.3,80.14 | v99.31,82.68 R105.2 97.88,83.48 97.54,83.82 97.03,83.82 94.74,86.11 94.74,87.12 93.73,88.14 92.71,88.14 91.44,86.87 91.44,86.04
  Top 0.559: 88.35,80.99 87.92,80.55 SJ54.2 86.87,80.75 | R107.2 88.35,80.99 | 88.35,80.99 88.35,81.75 88.56,81.95 C80.1 88.56,83.73 90.86,86.04 91.44,86.04 U27.8
  Top 0.762: 86.87,80.75 v86.87,82.04 v86.87,83.06
  Bottom 0.305: v99.31,82.68 99.31,81.15 v98.3,80.14
  Bottom 0.762: v86.87,83.06 v86.87,82.04 86.87,81.28 91.95,76.2 JP27.3
VCC27  (via drill 0.38)
  Top 0.305: SJ55.2 v114.05,80.14 | v115.06,82.68 R109.2 113.63,83.48 113.28,83.82 112.78,83.82 110.49,86.11 110.49,87.12 109.47,88.14 108.46,88.14 107.19,86.87 107.19,86.04
  Top 0.559: 104.1,80.99 103.66,80.55 SJ56.2 102.62,80.75 | R111.2 104.1,80.99 | 104.1,80.99 104.1,81.75 104.31,81.95 C83.1 104.31,83.73 106.61,86.04 107.19,86.04 U28.8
